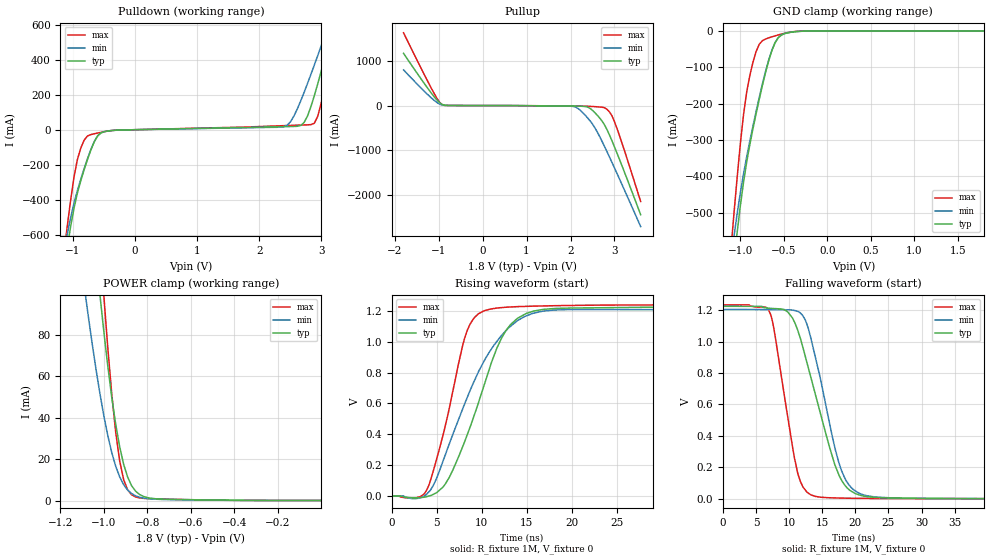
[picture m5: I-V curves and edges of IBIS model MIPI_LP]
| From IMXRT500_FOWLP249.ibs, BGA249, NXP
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[Model] MIPI_LP
Model_type   I/O
Polarity   Non-Inverting
Enable   Active-High
Vinh =   0.88
Vinl =   0.55
Vmeas = 0.6
Rref = 1M
Vref = 0
|   typ   min   max
C_comp  6.36p   6.29p   6.40p
[Temperature Range]   85   125   -40
[Voltage Range]   1.8   1.52   1.98
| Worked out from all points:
|   slope of the pulldown table from 0 to 0.27 V, typ, clamps not added: 135 ohm
|   slope of the pullup table from 0 to 0.27 V, typ, clamps not added: 15 kohm
|   GND clamp passes 1 mA (typ) near -0.32 V on its own axis
|   POWER clamp passes 1 mA (typ) near -0.78 V on its own axis
|   falling waveform, R_fixture 1M, V_fixture 0: 20-80 % time 4.73ns typ, 3.82ns min, 2.8ns max; typ from 1.23 V to 0 V
|   rising waveform, R_fixture 1M, V_fixture 0: 20-80 % time 4.51ns typ, 5.44ns min, 2.91ns max; typ from 0 V to 1.23 V
[GND_clamp]
|Voltage   I (typ)   I (min)   I (max)
-1.8V     -2.465A    -2.105A    -2.739A
-1.109V   -713.7mA   -632.1mA   -604.8mA
-1.073V   -631.9mA   -565.4mA   -502mA
-1.036V   -554.2mA   -502.9mA   -403.4mA
-963.7mV  -417.6mA   -394mA     -231.6mA
-927.4mV  -361.8mA   -347.2mA   -169.1mA
-818.3mV  -227.5mA   -221.2mA   -56.37mA
-745.6mV  -149.4mA   -145.3mA   -26.52mA
-672.8mV  -81.15mA   -79.28mA   -18.73mA
-600.1mV  -32.11mA   -32.03mA   -13.25mA
-454.7mV  -4.969mA   -4.378mA   -4.395mA
1.8V      27.05uA    49.33uA    10.62uA
[Power_clamp]
|Volatge   I (typ)   I (min)   I (max)
-1.8V     1.169A     796.8mA    1.63A
-1.091V   181.3mA    104mA      247.2mA
-1.073V   159.7mA    89.82mA    215.5mA
-1.018V   99.42mA    51.6mA     125.7mA
-1V       81.35mA    40.79mA    98.51mA
-963.7mV  49.68mA    23.11mA    51.21mA
-945.5mV  36.65mA    16.49mA    32.78mA
-927.4mV  25.88mA    11.38mA    18.99mA
-891mV    11.36mA    5.082mA    5.159mA
-854.6mV  4.549mA    2.295mA    1.73mA
-745.6mV  748uA      559uA      757.1uA
-180uV    27.07uA    17.18uA    17.66uA
[Pulldown]
|Volatge   I (typ)   I (min)   I (max)
-1.8V     -2.465A    -2.105A    -2.739A
-1.146V   -799.7mA   -703mA     -712mA
-1.037V   -555.7mA   -504.2mA   -405.5mA
-928mV    -363.2mA   -348.5mA   -171.1mA
-710mV    -115.8mA   -112.7mA   -27.83mA
-383mV    -5.267mA   -4.706mA   -4.937mA
2.397V    17.35mA    16.93mA    23.09mA
2.724V    41.4mA     213.4mA    27.19mA
2.887V    193.2mA    368.6mA    36.62mA
3.105V    477.6mA    587mA      334mA
3.268V    705.9mA    755.2mA    641.3mA
3.595V    1.178A     1.096A     1.284A
[Pullup]
|Volatge   I (typ)   I (min)   I (max)
-1.8V     1.173A     800.8mA    1.634A
-1.146V   252.2mA    152.5mA    349mA
-928mV    28.17mA    13.49mA    21.27mA
1.906V    -9.624mA   -10.35mA   -10mA
2.179V    -13.23mA   -71.58mA   -12.27mA
2.397V    -38.04mA   -287.6mA   -16.27mA
2.506V    -113.5mA   -425mA     -21.84mA
2.724V    -357.6mA   -817.6mA   -38.25mA
2.887V    -664.2mA   -1.159A    -144.4mA
2.996V    -919.7mA   -1.393A    -352.1mA
3.105V    -1.189A    -1.631A    -651.3mA
3.595V    -2.453A    -2.72A     -2.157A
[Ramp]
|variable   typ   min   max
dV/dt_r   744m/4.57n   735m/5.49n   750m/2.96n
dV/dt_f   744m/4.79n   736m/3.91n   750m/2.85n
R_load  = 1M
[Falling waveform]
R_fixture = 1M
V_fixture = 0
|time   V (typ)   V (min)   V (max)
0s        1.225V     1.205V     1.234V
6.9ns     1.213V     1.204V     1.202V
7.7ns     1.211V     1.204V     1.082V
9.8ns     1.189V     1.203V     517.7mV
11.2ns    1.084V     1.194V     180.7mV
12.4ns    912.4mV    1.142V     57.31mV
13.2ns    783mV      1.037V     26.47mV
17.3ns    174.4mV    261mV      4.327mV
19.8ns    37.57mV    55.22mV    2.459mV
50ns      131.9uV    172.3uV    18.82uV
[Rising waveform]
R_fixture = 1M
V_fixture = 0
|time   V (typ)   V (min)   V (max)
0s        -6.605uV   -3.333uV   7.253uV
2.7ns     -12.03mV   -17mV      -11.26mV
3.9ns     -4.081mV   12.12mV    39.67mV
5.9ns     72.55mV    258mV      439.7mV
8.1ns     349.7mV    595.1mV    1.02V
9.1ns     509.3mV    734.7mV    1.148V
10.3ns    723.5mV    877.6mV    1.2V
12.7ns    1.071V     1.071V     1.223V
15.8ns    1.198V     1.185V     1.23V
50ns      1.229V     1.207V     1.236V
